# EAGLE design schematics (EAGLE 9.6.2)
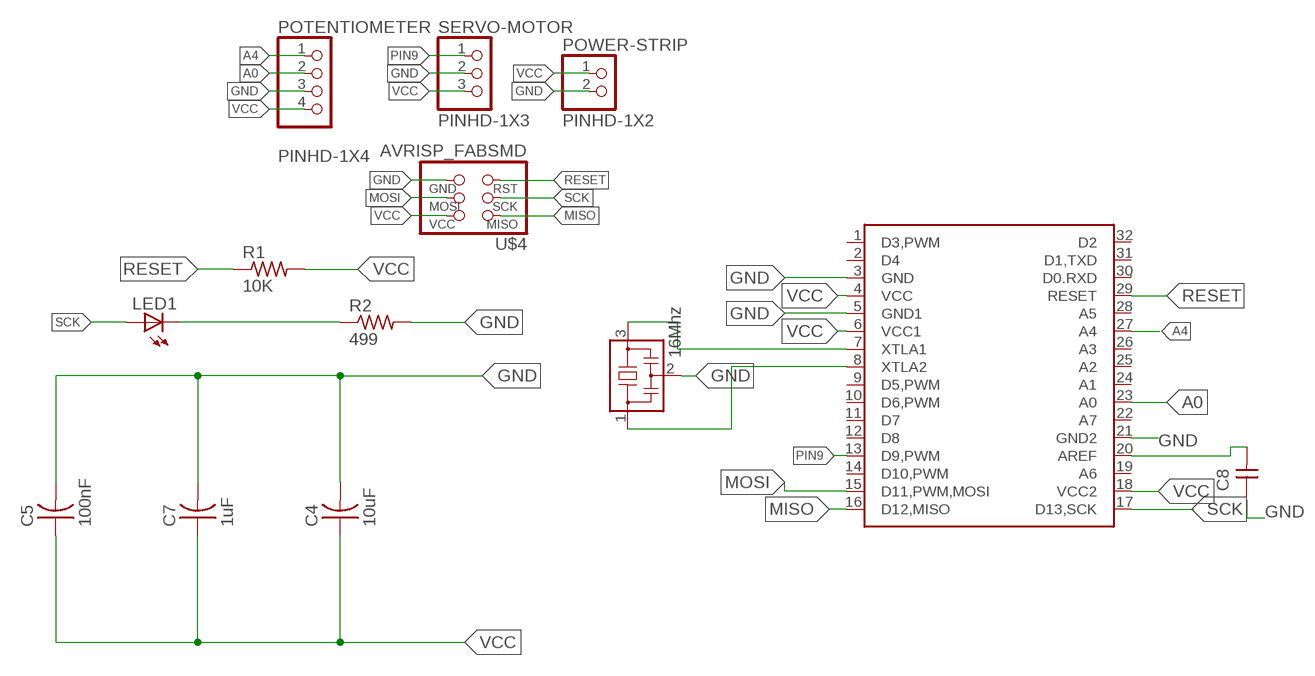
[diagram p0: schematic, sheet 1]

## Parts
C4  10uF  CAP-US1206FAB  [C1206FAB]
C5  100nF  CAP-US1206FAB  [C1206FAB]
C7  1uF  CAP-US1206FAB  [C1206FAB]
C8  CAP-UNPOLARIZEDFAB  [C1206FAB]
LED1  LEDSMT1206  [1206]
POTENTIOMETER  PINHD-1X4  [1X04]
POWER-STRIP  PINHD-1X2  [1X02]
R1  10K  RES-US1206FAB  [R1206FAB]
R2  499  MCS1632R050FER  [RES_1206]
RESONATOR1  16Mhz  RESONATOR  [EFOBM]
SERVO-MOTOR  PINHD-1X3  [1X03]
U$1  ATMEGA328P_TQFP_FAB.03  [QFP80P900X900X120-32L]
U$4  AVRISP_FABSMD  [2X03SMD]

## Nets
A0: POTENTIOMETER.2 U$1.23(A0)
A4: POTENTIOMETER.1 U$1.27(A4)
GND: C4.2 C5.2 C7.2 C8.1 POTENTIOMETER.3 POWER-STRIP.2 R2.2 RESONATOR1.2 SERVO-MOTOR.2 U$1.3(GND) U$1.5(GND1) U$1.21(GND2) U$4.6(GND)
MISO: U$1.16(D12,MISO) U$4.1(MISO)
MOSI: U$1.15(D11,PWM,MOSI) U$4.4(MOSI)
N$1: RESONATOR1.3 U$1.7(XTLA1)
N$5: RESONATOR1.1 U$1.8(XTLA2)
N$7: C8.2 U$1.20(AREF)
N$8: LED1.C R2.1
PIN9: SERVO-MOTOR.1 U$1.13(D9,PWM)
RESET: R1.1 U$1.29(RESET) U$4.5(RST)
RXD: U$1.30(D0.RXD)
SCK: LED1.A U$1.17(D13,SCK) U$4.3(SCK)
VCC: C4.1 C5.1 C7.1 POTENTIOMETER.4 POWER-STRIP.1 R1.2 SERVO-MOTOR.3 U$1.4(VCC) U$1.6(VCC1) U$1.18(VCC2) U$4.2(VCC)
Unconnected: U$1.1(D3,PWM) U$1.2(D4) U$1.9(D5,PWM) U$1.10(D6,PWM) U$1.11(D7) U$1.12(D8) U$1.14(D10,PWM) U$1.19(A6) U$1.22(A7) U$1.24(A1) U$1.25(A2) U$1.26(A3) U$1.28(A5) U$1.31(D1,TXD) U$1.32(D2)

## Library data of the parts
C4 C5 C7 = fab:CAP-US
C8 = fab:CAP-UNPOLARIZED
LED1 = adafruit:LED: LED
POTENTIOMETER = Connector:PINHD-1X4: PIN HEADER; CATEGORY: CONNECTOR; SUB-CATEGORY: PIN-HEADER
POWER-STRIP = Connector:PINHD-1X2: PIN HEADER; CATEGORY: CONNECTOR; SUB-CATEGORY: PIN-HEADER
R1 = fab:RES-US: Resistor (US Symbol)
R2 = Resistor_Capacitor:MCS1632R050FER: RES 0.05 OHM 1% 1W 1632; CREATED_BY: PCBLayout.com; DIGIKEY_PART_NUMBER: MCS1632R050FERTR-ND; MANUFACTURER: Ohmite; MPN: MCS1632R050FER; PACKAGE: SMD 1206
RESONATOR1 = fab:RESONATOR
SERVO-MOTOR = Connector:PINHD-1X3: PIN HEADER; CATEGORY: CONNECTOR; SUB-CATEGORY: PIN-HEADER
U$1 = fablab:ATMEGA328P_TQFP_FAB.03
U$4 = fablab (1):AVRISP_FAB

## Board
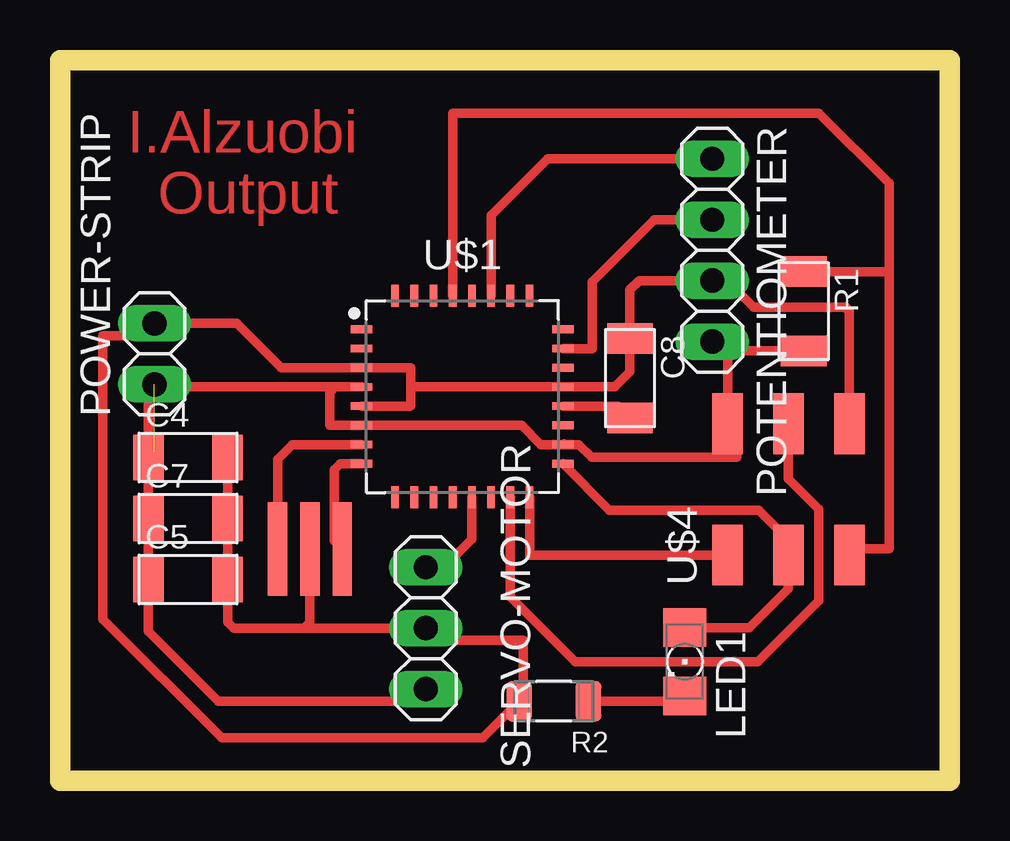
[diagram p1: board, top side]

Size 37.06 x 30.02 mm. Coordinates in mm from the lower left corner, seen from the top.
Outline: 0,0 37.06,0 37.06,30.02 0,30.02 0,0
Copper layers (1*16): Top 0.035mm / dielectric 1.5mm / Bottom 0.035mm
Design rules "default *": minimum track width 0.4mm, minimum drill 0.35mm, track to track 0.4mm, track to pad 0.4mm, pad to pad 0.4mm, via to via 0.4mm, smd to smd 0.4mm, copper to edge 40mil, drill to drill 6mil, minimum pad ring 10mil, minimum via ring 8mil, stop-mask expansion 4mil, vias tented up to drill 0mil, thermal gap 10mil

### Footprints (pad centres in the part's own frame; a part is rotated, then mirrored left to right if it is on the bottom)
C1206FAB = smd 1.27 x 1.905: 1 -1.651,0; 2 1.651,0
1206 = smd 1.6 x 1.803: A -1.422,0; C 1.422,0
1X04 = drill 1.016 long: 1 -3.81,0; 2 -1.27,0; 3 1.27,0; 4 3.81,0
1X02 = drill 1.016 long: 1 -1.27,0; 2 1.27,0
R1206FAB = smd 1.27 x 1.905: 1 -1.651,0; 2 1.651,0
RES_1206 = smd 1.08 x 1.68: 1 -1.445,0; 2 1.445,0
EFOBM = smd 0.8 x 3.9: 1 -1.35,0; 2 0,0; 3 1.35,0
1X03 = drill 1.016 long: 1 -2.54,0; 2 0,0; 3 2.54,0
QFP80P900X900X120-32L = smd 0.906 x 0.32: 1 -4.197,2.8; 2 -4.197,2; 3 -4.197,1.2; 4 -4.197,0.4; 5 -4.197,-0.4; 6 -4.197,-1.2; 7 -4.197,-2; 8 -4.197,-2.8; 17 4.197,-2.8; 18 4.197,-2; 19 4.197,-1.2; 20 4.197,-0.4; 21 4.197,0.4; 22 4.197,1.2; 23 4.197,2; 24 4.197,2.8 | smd 0.32 x 0.906: 9 -2.8,-4.197; 10 -2,-4.197; 11 -1.2,-4.197; 12 -0.4,-4.197; 13 0.4,-4.197; 14 1.2,-4.197; 15 2,-4.197; 16 2.8,-4.197; 25 2.8,4.197; 26 2,4.197; 27 1.2,4.197; 28 0.4,4.197; 29 -0.4,4.197; 30 -1.2,4.197; 31 -2,4.197; 32 -2.8,4.197
2X03SMD = smd 2.54 x 1.27: 1 -2.54,2.54; 2 2.92,2.54; 3 -2.54,0; 4 2.92,0; 5 -2.54,-2.54; 6 2.92,-2.54

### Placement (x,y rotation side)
C4  5.33,13.46 0 top
C5  5.33,8.38 0 top
C7  5.33,10.92 0 top
C8  23.75,16.76 270 top
LED1  26.04,4.95 270 top
POTENTIOMETER  27.18,22.1 270 top
POWER-STRIP  3.94,17.78 90 top
R1  30.99,19.56 270 top
R2  20.57,3.3 180 top
RESONATOR1  10.41,9.65 180 top
SERVO-MOTOR  15.24,6.35 270 top
U$1  16.76,16 0 top
U$4  30.35,11.94 90 top

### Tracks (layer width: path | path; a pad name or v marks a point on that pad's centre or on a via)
A0
  Top 0.4: U$1.23 22.19,18 22.19,20.79 24.76,23.37 POTENTIOMETER.2
A4
  Top 0.4: U$1.27 17.96,23.55 20.32,25.91 POTENTIOMETER.1
GND
  Top 0.4: 14.61,16.38 14.62,16.4 U$1.21 23.11,16.4 23.75,17.04 C8.1 23.75,20.45 24.13,20.83 POTENTIOMETER.3 | 14.61,16.38 14.61,15.62 14.59,15.6 U$1.5 | 14.61,16.38 14.61,17.2 U$1.3 9.21,17.2 7.37,19.05 POWER-STRIP.2 3.43,18.54 1.78,18.54 1.78,6.73 6.73,1.78 17.61,1.78 R2.2 19.3,3.48 19.3,5.84 15.75,5.84 SERVO-MOTOR.2 10.16,6.35 | RESONATOR1.2 10.41,6.6 10.16,6.35 | 10.16,6.35 7.24,6.35 6.98,6.6 C5.2 C7.2 C4.2 | U$4.6 32.89,19.56 32.73,19.72 28.9,19.72 27.79,20.83 POTENTIOMETER.3 | 26.04,20.83 POTENTIOMETER.3
MISO
  Top 0.4: U$4.1 19.56,9.4 U$1.16
MOSI
  Top 0.4: U$1.15 18.76,7.65 21.46,4.95 29.08,4.95 31.62,7.49 31.62,11.3 30.35,12.57 U$4.4
N$1
  Top 0.4: U$1.7 9.68,14 9.06,13.38 RESONATOR1.3
N$5
  Top 0.4: U$1.8 11.68,13.2 11.43,12.95 11.43,9.99 RESONATOR1.1
N$7
  Top 0.4: U$1.20 23.26,15.6 C8.2
N$8
  Top 0.4: LED1.C 25.81,3.3 R2.1
PIN9
  Top 0.4: U$1.13 17.16,10.05 16,8.89 SERVO-MOTOR.1
RESET
  Top 0.4: U$1.29 16.36,27.81 31.62,27.81 34.54,24.89 34.54,21.21 | U$4.5 33.15,9.65 34.54,9.65 34.54,21.21 | 34.54,21.21 R1.1
SCK
  Top 0.4: U$1.17 22.89,11.27 29.12,11.27 30.35,10.03 U$4.3 30.35,8 28.73,6.38 LED1.A
VCC  (1 unrouted)
  Top 0.4: U$1.18 20.03,14 19.23,14.8 U$1.6 11.23,14.8 11.23,16.19 11.45,16.4 | 11.45,16.4 U$1.4 | U$1.18 21,14.04 | 27.81,14 27.81,14.73 | 27.81,14.73 U$4.2 | 27.69,14.98 U$4.2 | C4.1 C7.1 C5.1 3.68,6.22 6.6,3.3 14.73,3.3 SERVO-MOTOR.3 | U$1.18 21.62,14 22.16,13.46 28.19,13.46 28.19,14.48 U$4.2 | 28.19,15.11 27.81,14.73 | U$4.2 27.81,17.65 27.56,17.91 | 27.56,17.91 POTENTIOMETER.4 | R1.2 27.56,17.91 | C4.1 3.94,13.72 | 11.45,16.4 4.04,16.4 3.68,16.04 C4.1

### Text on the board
Top: I.Alzuobi | Output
